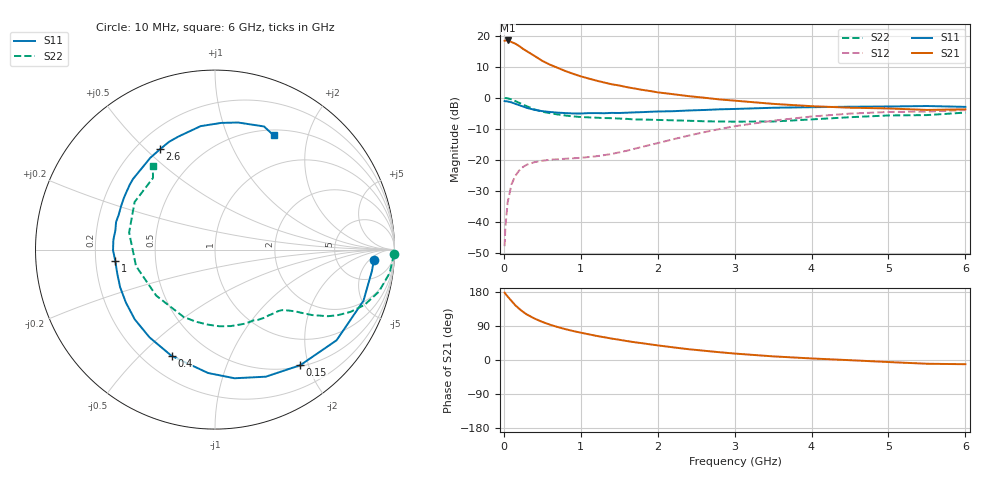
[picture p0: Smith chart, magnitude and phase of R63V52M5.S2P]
! SIEMENS Small Signal Semiconductors
! BFR193
! Si NPN RF Bipolar Junction Transistor in SOT23
! VCE = 3.5 V  IC = 2.5 mA
! Common Emitter S-Parameters:  May  1996
# GHz  S  MA  R  50
!  f  S11  S21  S12  S22
! GHz  MAG  ANG  MAG  ANG  MAG  ANG  MAG  ANG
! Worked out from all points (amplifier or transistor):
!   36 points, 10 MHz to 6 GHz, reference 50 ohm
!   highest |S21| = 18.5 dB at 50 MHz (marker M1)
!   |S21| within 3 dB of that: start of sweep to 268.4 MHz
!   unconditionally stable (mu >= 1): 1.112 GHz to 2.033 GHz
!   at 250 MHz: K = 0.27, MSG = 19.0 dB, |S12| = -22.2 dB
!   at 1.4 GHz: K = 1.10, MAG = 9.3 dB, |S12| = -18.1 dB
!   at 6 GHz: K = 0.99, MSG = 0.1 dB, |S12| = -3.9 dB
!   S11 on the Smith chart (normalised r, x): 10 MHz: 13, -7; 150 MHz: 0.52, -1.87; 400 MHz: 0.31, -0.63; 1 GHz: 0.28, -0.05; 2.6 GHz: 0.29, +0.55; 6 GHz: 0.57, +1.48
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0.01  0.8867 -3.9  8.291 177.8  0.0041 86.7  0.9967 -1.5
0.02  0.8825 -7.7  8.364 174.8  0.0083 85.0  0.9922 -3.0
0.05  0.8749 -19.0  8.386 167.4  0.021 80.0  0.982 -7.6
0.1  0.8451 -36.7  7.912 155.8  0.0406 70.9  0.9426 -14.4
0.15  0.8003 -53.6  7.431 144.2  0.0558 62.5  0.8882 -20.3
0.2  0.7626 -68.2  6.809 135.1  0.0678 56.0  0.8308 -24.7
0.25  0.725 -81.4  6.131 127.0  0.0773 50.6  0.7772 -28.0
0.3  0.6887 -93.2  5.617 120.0  0.0842 46.6  0.7313 -30.5
0.4  0.6397 -112.2  4.72 109.3  0.0924 41.1  0.6522 -34.0
0.5  0.6101 -126.7  3.933 100.5  0.0972 38.0  0.5986 -36.1
0.6  0.5925 -139.0  3.42 93.2  0.1009 36.3  0.5661 -37.5
0.8  0.5686 -158.4  2.701 81.4  0.1047 37.1  0.5195 -40.6
1  0.5591 -173.3  2.216 72.1  0.1084 41.1  0.492 -44.1
1.1  0.5681 -179.7  2.05 67.9  0.1114 43.4  0.485 -46.3
1.4  0.5722 164.4  1.656 56.6  0.1249 51.2  0.4707 -53.4
1.6  0.5767 155.1  1.485 50.0  0.141 56.0  0.4584 -58.8
2.2  0.6096 132.1  1.145 33.4  0.2153 61.8  0.4349 -78.5
2.6  0.6373 118.8  1.006 24.5  0.2794 59.5  0.4201 -95.1
3.5  0.6926 96.6  0.8 9.6  0.4288 45.1  0.416 -142.0
4.5  0.7196 79.7  0.694 -0.5  0.5574 25.3  0.4879 168.7
5.5  0.7384 68.3  0.639 -9.9  0.6011 6.4  0.5277 130.9
6  0.7158 62.9  0.653 -11.1  0.6357 1.2  0.5792 126.7
